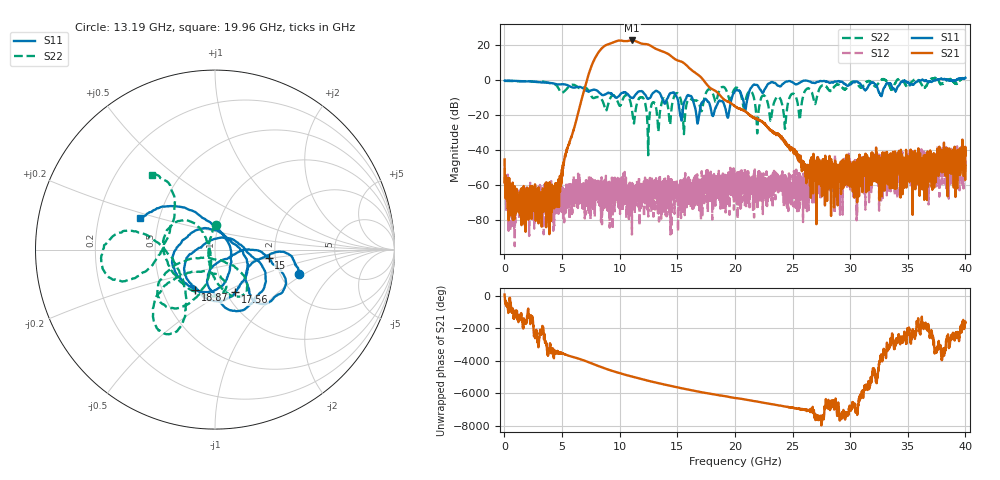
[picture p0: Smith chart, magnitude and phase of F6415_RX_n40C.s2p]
!Keysight Technologies,N5245B,MY52451815,A.15.70.20
!Date: Wednesday, April 17, 2024 15:41:16
!Correction: S33(C  2-Port  )
!S43(C  2-Port  )
!S34(C  2-Port  )
!S44(C  2-Port  )
!S2P File: Measurements: S33, S43, S34, S44:
# Hz S  RI  R 50
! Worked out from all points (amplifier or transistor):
!   4000 points, 10 MHz to 40 GHz, reference 50 ohm
!   highest |S21| = 22.5 dB at 11.08 GHz (marker M1)
!   |S21| within 3 dB of that: 8.714 GHz to 12.68 GHz (3.966 GHz wide, 37.1 % of centre)
!   unconditionally stable (mu >= 1): start of sweep to 32.7 GHz; 33.06 GHz to 34.07 GHz; 34.48 GHz to 35.52 GHz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
!   at 6.67 GHz: K = 2426.46, MAG = -7.8 dB, |S12| = -69.8 dB
!   at 20.01 GHz: K = 1274.49, MAG = -12.2 dB, |S12| = -58.8 dB
!   at 40 GHz: K = 582.63, MSG = 0.5 dB, |S12| = -43.9 dB
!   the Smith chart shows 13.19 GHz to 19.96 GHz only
!   S11 on the Smith chart (normalised r, x): 13.19 GHz: 2.55, -0.90; 15 GHz: 1.84, -0.19; 17.56 GHz: 1.10, -0.56; 18.87 GHz: 0.73, -0.35; 19.96 GHz: 0.39, +0.17
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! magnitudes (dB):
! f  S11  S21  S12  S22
! 10 MHz  -0.4  -45.4  -50.6  -0.6
! 760 MHz  -0.5  -61.9  -67.2  -0.7
! 4.2 GHz  -1.9  -70.1  -69.1  -2.2
! 6.68 GHz  -4.3  -11.4  -67.9  -4.7
! 8.34 GHz  -7.9  17.3  -62.5  -10.3
! 11.08 GHz  -10.2  22.5  -58.8  -18.0
! 13.19 GHz  -6.2  17.6  -61.1  -17.1
! 13.34 GHz  -6.8  17.2  -56.8  -28.4
! 15 GHz  -10.4  11.2  -61.4  -7.6
! 15.59 GHz  -12.7  9.5  -60.2  -29.1
! 17.56 GHz  -11.6  -2.6  -56.2  -6.5
! 18.87 GHz  -12.0  -10.0  -73.9  -4.1
! 19.39 GHz  -21.5  -12.4  -61.2  -8.4
! 19.96 GHz  -6.9  -14.9  -54.6  -5.2
! 20.01 GHz  -6.4  -15.1  -58.8  -4.8
! 23.8 GHz  -3.4  -31.4  -57.6  -9.9
! 24.34 GHz  -1.4  -35.3  -65.4  -27.9
! 24.92 GHz  -1.1  -39.6  -60.3  -8.1
! 25.62 GHz  -1.6  -44.1  -55.8  -22.7
! 26.67 GHz  -1.6  -54.1  -48.9  -7.0
! 33.34 GHz  -2.2  -43.9  -63.1  -2.5
! 40 GHz  1.2  -43.0  -43.9  0.6
